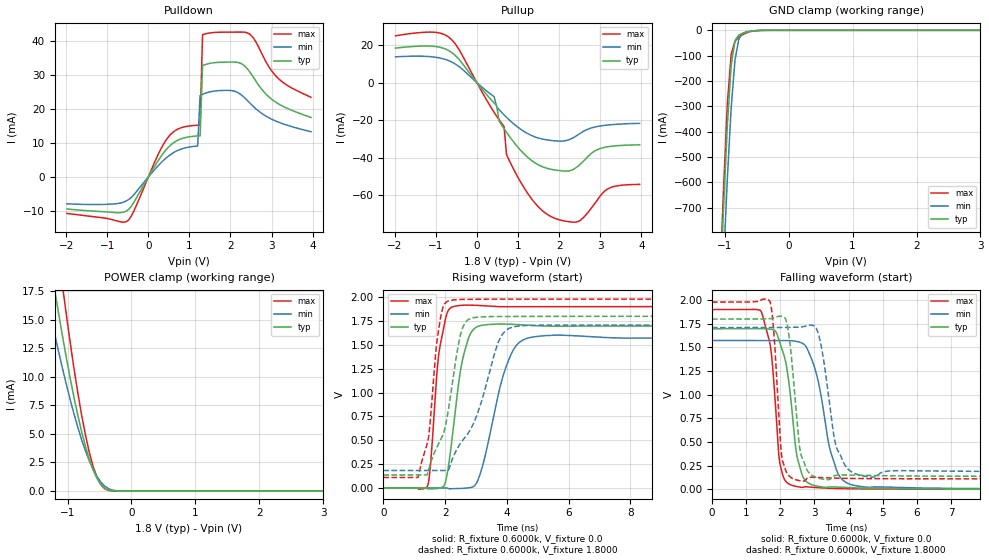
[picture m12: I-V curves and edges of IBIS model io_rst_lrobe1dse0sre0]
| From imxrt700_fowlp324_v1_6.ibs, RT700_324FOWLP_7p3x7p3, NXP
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[Model] io_rst_lrobe1dse0sre0
|   Model io_rst_lrobe1dse0sre0
| This model was characterised for following simulation conditions:
| External (pad) voltage:
|   - Typ: 1.8V,   - Min: 1.71V,   - Max: 1.98V
| Library cells for typ/min/max conditions are connected as defined below:
|  PAD_RST - External Pad
|  ipp_do - Core Input
|  ipp_obe - Output Buffer Enable
|  ASRCN3V3[3] - NC
|  ASRCN3V3[4] - NC
|  ASRCP3V3[4] - NC
|  REFAPBIAS3V3 - gnde
|  REFBAMPL3V3 - vdd1v8
|  REFCAMPH3V3 - vdd1v8
|  REFDNBIAS3V3 - vdd1v8
|  REFH3V3 - REFH3V3
|  REFL3V3 - REFL3V3
|  gnde - gnde
|  ipp_dse - gnde
|  ipp_ina235_3v - NC
|  ipp_ina40_3v - NC
|  ipp_ina_mux - NC
|  ipp_ind - NC
|  ipp_ind_1p8v - NC
|  ipp_ind_3v - NC
|  ipp_sre - gnde
|  vdd - vdd
|  vdd1v8 - vdd1v8
|  vdda - vdde3v3
|  vdde3v3 - vdde3v3
| All other pins connected to ground
Model_type I/O
Polarity   Non-Inverting
Enable   Active-High
Vinl =   0.5400V
Vinh =   1.2600V
Vmeas =  0.9000V
Cref =   15.0000pF
Rref =   0.6000k
Vref =   0.0V
C_comp   3.9805pF   3.7965pF   4.1056pF
|C_comp_pullup   0.3209pF   0.4282pF   0.2792pF
|C_comp_pulldown   2.2500pF   2.3235pF   2.0512pF
[Model Spec]
| variable   typ   min   max
Vinh   1.2600V   NA   NA
Vinl   0.5400V   NA   NA
Vref   0.0V   0.0V   0.0V
Cref   15.0000pF   15.0000pF   15.0000pF
Rref   0.6000k   0.6000k   0.6000k
[Receiver Thresholds]
Vcross_high  =   0.0V
Vcross_low  =   0.0V
Vdiff_ac  =   0.0V
Vdiff_dc  =   0.0V
Tdiffslew_ac  =   0.0S
[Temperature Range]   25.0000   0.1250k   -40.0000
[Voltage Range]   1.8000V   1.7100V   1.9800V
[Pullup Reference]   1.8000V   1.7100V   1.9800V
[Pulldown Reference]   0.0V   0.0V   0.0V
[POWER Clamp Reference]   1.8000V   1.7100V   1.9800V
[GND Clamp Reference]   0.0V   0.0V   0.0V
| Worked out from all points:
|   slope of the pulldown table from 0 to 0.27 V, typ, clamps not added: 50.4 ohm
|   slope of the pullup table from 0 to 0.27 V, typ, clamps not added: 37.3 ohm
|   GND clamp passes 1 mA (typ) near -0.50 V on its own axis
|   POWER clamp passes 1 mA (typ) near -0.53 V on its own axis
|   rising waveform, R_fixture 0.6000k, V_fixture 0.0: 20-80 % time 416ps typ, 681ps min, 294ps max; typ from 0 V to 1.7 V
|   rising waveform, R_fixture 0.6000k, V_fixture 1.8000: 20-80 % time 612ps typ, 1.05ns min, 327ps max; typ from 0.135 V to 1.8 V
|   falling waveform, R_fixture 0.6000k, V_fixture 0.0: 20-80 % time 342ps typ, 520ps min, 245ps max; typ from 1.7 V to 0 V
|   falling waveform, R_fixture 0.6000k, V_fixture 1.8000: 20-80 % time 249ps typ, 359ps min, 185ps max; typ from 1.8 V to 0.135 V
[Pulldown]
|Voltage   I(typ)   I(min)   I(max)
-1.98V    -9.436mA   -7.895mA   -10.73mA
-480mV    -9.541mA   -6.639mA   -12.66mA
480mV     8.648mA    6.047mA    11.65mA
780mV     11.14mA    8.115mA    14.39mA
1.2V      12.06mA    9.106mA    15.21mA
1.26V     12.11mA    23.95mA    15.25mA
1.32V     32.75mA    24.3mA     41.84mA
2.04V     33.78mA    25.37mA    42.6mA
2.46V     31.05mA    21.89mA    42.07mA
2.82V     24.92mA    18.22mA    34.85mA
3.12V     21.84mA    16.35mA    29.49mA
3.96V     17.49mA    13.29mA    23.43mA
[Pullup]
|Voltage   I(typ)   I(min)   I(max)
-1.98V    18.49mA    13.82mA    25.02mA
-960mV    19.18mA    13.43mA    26.78mA
-540mV    14.81mA    10.16mA    21.1mA
480mV     -12.23mA   -12.98mA   -17.88mA
540mV     -20.55mA   -14.43mA   -19.82mA
660mV     -24.59mA   -17.2mA    -23.43mA
720mV     -26.52mA   -18.51mA   -38.45mA
960mV     -33.51mA   -23.18mA   -49.04mA
1.74V     -45.96mA   -30.69mA   -70.78mA
2.46V     -44.61mA   -27.85mA   -74.24mA
3.18V     -34.28mA   -22.63mA   -56.83mA
3.96V     -33.2mA    -21.72mA   -54.36mA
[GND_clamp]
|Voltage   I(typ)   I(min)   I(max)
-1.98V    -7.543A    -7.6A      -7.897A
-1.08V    -1.077A    -1.286A    -1.025A
-1.02V    -705.3mA   -921.3mA   -628.8mA
-960mV    -377.1mA   -587.4mA   -291.7mA
-900mV    -139.2mA   -307mA     -94.38mA
-840mV    -40.12mA   -117mA     -42.82mA
-780mV    -18.81mA   -33.95mA   -26.13mA
-720mV    -11.86mA   -11.44mA   -16.78mA
-660mV    -7.061mA   -5.737mA   -9.992mA
-540mV    -1.684mA   -1.901mA   -2.15mA
-420mV    -207.1uA   -403.7uA   -160.6uA
3.96V     0A         0A         0A
[POWER_clamp]
|Voltage   I(typ)   I(min)   I(max)
-1.98V    46.79mA    35.95mA    61.44mA
-1.32V    21.78mA    16.85mA    28.96mA
-1.2V     17.57mA    13.71mA    23.37mA
-1.08V    13.59mA    10.75mA    18.03mA
-1.02V    11.71mA    9.354mA    15.49mA
-900mV    8.21mA     6.76mA     10.75mA
-720mV    3.899mA    3.511mA    4.896mA
-600mV    1.839mA    1.889mA    2.143mA
-540mV    1.103mA    1.267mA    1.197mA
-420mV    244.5uA    429.3uA    190.7uA
-180mV    281nA      5.273uA    27.6nA
3.96V     0A         0A         0A
[Ramp]
| variable   typ   min   max
dV/dt_r  1.0188/0.4161n   0.9441/0.6811n   1.1406/0.2939n
dV/dt_f  0.9990/0.2493n   0.9166/0.3588n   1.1224/0.1850n
R_load = 0.6000k
[Rising Waveform]
R_fixture= 0.6000k
V_fixture= 0.0
V_fixture_min= 0.0
V_fixture_max= 0.0
|time   V(typ)   V(min)   V(max)
0s        119.2nV    3.183uV    128.2nV
1.428ns   -8.641mV   -709.1uV   17.87mV
1.522ns   -9.674mV   -1.023mV   224.9mV
1.825ns   -1.493mV   -1.059mV   1.469V
2.062ns   136.8mV    -804.4uV   1.83V
2.448ns   1.125V     -6.145mV   1.912V
2.987ns   1.68V      36.49mV    1.915V
4.138ns   1.716V     1.402V     1.9V
5.12ns    1.698V     1.593V     1.9V
60ns      1.698V     1.573V     1.901V
[Rising Waveform]
R_fixture= 0.6000k
V_fixture= 1.8000
V_fixture_min= 1.7100
V_fixture_max= 1.9800
|time   V(typ)   V(min)   V(max)
0s        135mV      182.4mV    109.3mV
1.126ns   134.2mV    182.3mV    114.7mV
1.471ns   196.8mV    181.6mV    549.6mV
1.712ns   412.4mV    181.6mV    1.473V
1.87ns    514.2mV    181.9mV    1.817V
2.299ns   1.245V     351.2mV    1.972V
2.729ns   1.76V      565.6mV    1.977V
3.789ns   1.797V     1.575V     1.979V
4.479ns   1.798V     1.699V     1.979V
60ns      1.8V       1.71V      1.98V
[Falling Waveform]
R_fixture= 0.6000k
V_fixture= 0.0
V_fixture_min= 0.0
V_fixture_max= 0.0
|time   V(typ)   V(min)   V(max)
0s        1.698V     1.573V     1.901V
1.427ns   1.699V     1.573V     1.887V
1.709ns   1.694V     1.574V     1.517V
1.869ns   1.667V     1.573V     833.8mV
2.082ns   1.446V     1.574V     136.3mV
2.625ns   164.6mV    1.548V     18.6mV
3.048ns   33.86mV    1.236V     16.98mV
3.689ns   21.27mV    165.3mV    6.823mV
4.579ns   9.572mV    19.46mV    2.36mV
60ns      7.28uV     14.94uV    3.617uV
[Falling Waveform]
R_fixture= 0.6000k
V_fixture= 1.8000
V_fixture_min= 1.7100
V_fixture_max= 1.9800
|time   V(typ)   V(min)   V(max)
0s        1.8V       1.71V      1.98V
1.692ns   1.804V     1.71V      1.99V
1.796ns   1.809V     1.709V     1.728V
2.059ns   1.829V     1.71V      308.4mV
2.241ns   1.66V      1.712V     146.5mV
2.658ns   317.3mV    1.719V     84.43mV
3.127ns   115.4mV    1.63V      123.5mV
3.675ns   148mV      413.5mV    116.2mV
4.646ns   144mV      127.8mV    111.4mV
60ns      135mV      182.4mV    109.3mV
